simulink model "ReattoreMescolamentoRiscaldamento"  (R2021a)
settings: Solver=VariableStepAuto  StartTime=0.0  StopTime=200000  RelTol=1e-3
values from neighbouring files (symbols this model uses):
  Ke = 30    [scambiatoredicalore_dati.m]    (also in scambiatoremodelloTD.m)
undefined symbols (not defined in the file or in its folder): Am, c, cr, m, mr, Q, T0, Ti, Tr0, w

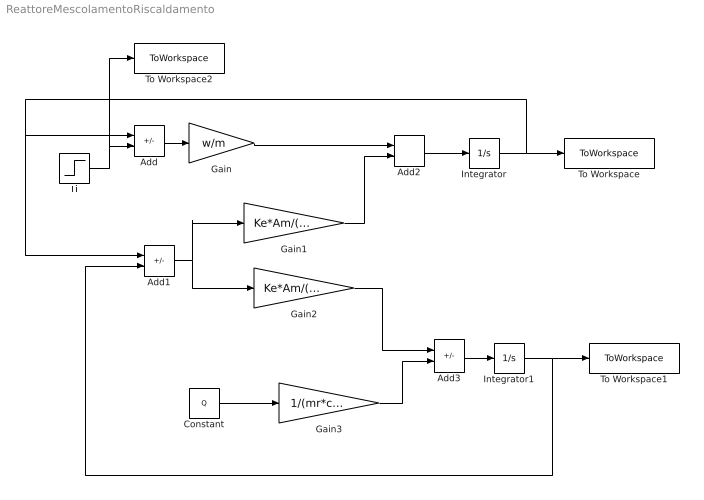
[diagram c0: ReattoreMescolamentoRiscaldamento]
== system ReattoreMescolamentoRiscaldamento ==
  Add : Sum  Inputs=-+
  Add1 : Sum  Inputs=-+
  Add2 : Sum
  Add3 : Sum  Inputs=-+
  Constant : Constant  Value=Q
  Gain : Gain  Gain=w/m
  Gain1 : Gain  Gain=Ke*Am/(m*c)
  Gain2 : Gain  Gain=Ke*Am/(mr*cr)
  Gain3 : Gain  Gain=1/(mr*cr)
  Integrator : Integrator  InitialCondition=T0
  Integrator1 : Integrator  InitialCondition=Tr0
  Ti : Step  Time=100000  Before=Ti  After=Ti+10  SampleTime=0
  To Workspace : ToWorkspace  VariableName=T_ws  SaveFormat=Timeseries  SampleTime=-1
  To Workspace1 : ToWorkspace  VariableName=Tr_ws  SaveFormat=Timeseries  SampleTime=-1
  To Workspace2 : ToWorkspace  VariableName=Ti_ws  SaveFormat=Timeseries  SampleTime=-1
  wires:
  Ti/1 -> To Workspace2/1, Add/2
  Integrator/1 -> To Workspace/1, Add/1, Add1/1
  Add/1 -> Gain/1
  Integrator1/1 -> To Workspace1/1, Add1/2
  Add1/1 -> Gain2/1, Gain1/1
  Gain/1 -> Add2/1
  Add2/1 -> Integrator/1
  Gain1/1 -> Add2/2
  Add3/1 -> Integrator1/1
  Gain2/1 -> Add3/1
  Gain3/1 -> Add3/2
  Constant/1 -> Gain3/1
